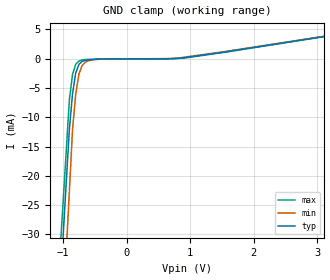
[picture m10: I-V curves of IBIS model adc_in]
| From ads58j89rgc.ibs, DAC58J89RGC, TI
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[Model] adc_in
Model_type Terminator
C_comp 1.37000pF 1.20000pF 1.54000pF
| variable typ   min   max
[Voltage Range] 1.90000V 1.80000V 2.00000V
[POWER Clamp Reference] 1.90000V 1.80000V 2.00000V
[GND Clamp Reference] 0.00000V 0.00000V 0.00000V
[Temperature Range]   25   85   -40
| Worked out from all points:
|   GND clamp passes 1 mA (typ) near -0.75 V on its own axis
[GND Clamp]
-1.9V     -198.3mA   -235.3mA   -184.9mA
-900mV    -12.06mA   -22.71mA   -7.056mA
-850mV    -5.966mA   -12.08mA   -2.68mA
-800mV    -2.467mA   -6.063mA   -947.5uA
-750mV    -983.8uA   -2.646mA   -399.4uA
-700mV    -459uA     -1.163mA   -214.5uA
-650mV    -307.9uA   -609.5uA   -139.9uA
-600mV    -156.9uA   -336.1uA   -121uA
-500mV    -109.4uA   -122.1uA   -83.19uA
600mV     4.767uA    3.684uA    2.028uA
900mV     179uA      257.7uA    103.1uA
3.8V      4.984mA    5mA        4.97mA
[POWER Clamp]
-1.9V     0A         0A         0A
3.8V      0A         0A         0A
